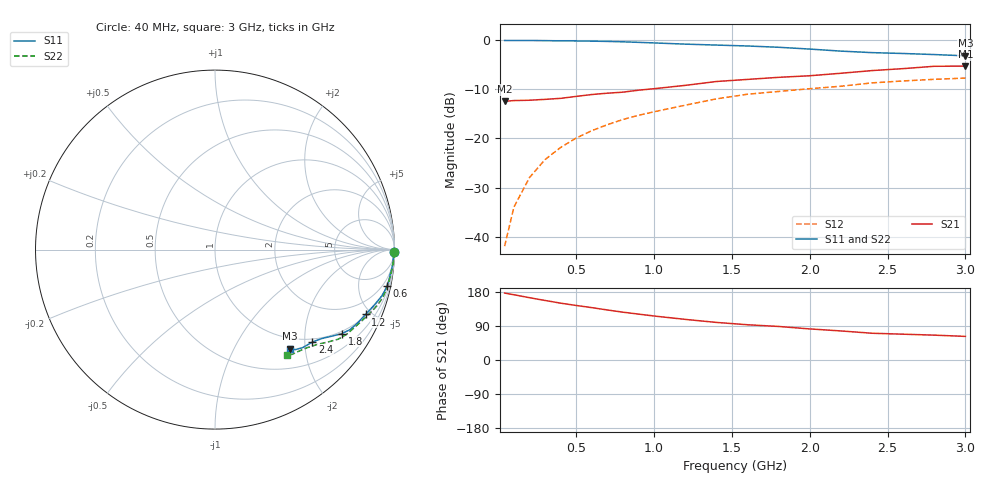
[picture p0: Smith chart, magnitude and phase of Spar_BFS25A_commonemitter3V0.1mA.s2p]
! Filename:  BFS25AF.S2P  Version:  4.0
! NXP part #: BFS25A  Date: Jun 1994
! Bias condition: Vce=3V, Ic=0.1mA
#  MHz  S  MA  R  50
! Freq  S11  S21  S12  S22  !GUM [dB]
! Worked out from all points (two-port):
!   21 points, 40 MHz to 3 GHz, reference 50 ohm
!   highest |S21| = -5.27 dB at 3 GHz (marker M1); lowest = -12.4 dB at 40 MHz (marker M2)
!   |S21| within 3 dB of the highest: 1.462 GHz to end of sweep
!   lowest |S11| = -3.2 dB at 3 GHz (marker M3), VSWR 5.54, Z = 40.3 - j86 ohm
!   |S11| at or under -10 dB: nowhere
!   |S22| runs from -3.0 to 0.0 dB; largest |S21 - S12| = 0.25
!   S11 on the Smith chart (normalised r, x): 40 MHz: open; 600 MHz: 0.98, -9.50; 1.2 GHz: 1.06, -4.62; 1.8 GHz: 0.92, -3.07; 2.4 GHz: 0.93, -2.17; 3 GHz: 0.81, -1.72
40  0.995 -0.8  0.239 176.6  0.008 89.0  0.999 -0.9
100  0.994 -1.8  0.243 172.2  0.02 86.6  0.999 -2.1
200  0.994 -3.9  0.245 164.4  0.04 84.5  0.995 -4.3
300  0.991 -5.9  0.25 157.1  0.061 82.0  0.992 -6.5
400  0.986 -7.9  0.256 150.0  0.081 80.3  0.988 -8.8
500  0.984 -9.9  0.268 143.9  0.101 78.6  0.984 -11.1
600  0.979 -11.9  0.28 138.2  0.12 76.9  0.979 -13.2
700  0.973 -13.8  0.289 132.0  0.138 75.3  0.974 -15.3
800  0.964 -15.6  0.296 126.2  0.156 73.3  0.966 -17.1
900  0.952 -17.3  0.31 121.1  0.172 71.1  0.955 -19.1
1000  0.939 -19.3  0.321 116.1  0.187 68.9  0.943 -20.9
1200  0.913 -23.3  0.347 107.2  0.218 64.3  0.915 -25.0
1400  0.893 -27.4  0.38 99.2  0.253 60.6  0.89 -29.2
1600  0.874 -30.7  0.399 93.0  0.282 57.0  0.872 -32.8
1800  0.848 -33.5  0.419 88.5  0.301 54.8  0.848 -36.1
2000  0.813 -36.3  0.435 82.0  0.321 51.2  0.815 -39.1
2200  0.775 -39.7  0.461 76.7  0.34 48.0  0.78 -42.5
2400  0.748 -43.5  0.491 70.6  0.368 44.3  0.751 -46.6
2600  0.733 -48.1  0.514 68.1  0.385 41.4  0.733 -50.7
2800  0.715 -51.2  0.543 65.6  0.4 40.5  0.725 -53.6
3000  0.694 -52.8  0.545 62.3  0.412 38.3  0.708 -55.7
